|   IBIS model for TI TMS320C6474 DSP
[IBIS Ver]   5.0
[Disclaimer]   Please be aware that in the absence of a written agreement
|   Texas Instruments(TI) assumes no liability for:
|   (1) The accuracy of the IBIS models provided to your company,
|   however, the IBIS model is compliant to industry standard
|   IQ Level 2a.  Refer to IBIS Quality Section below for
|   for full details.
|   (2) The proper functioning of these Models in your design
|   or for any resulting applications
|   (3) Infringement of patents, copyrights or intellectual
|   property rights resulting from your use of these
|   models.
|   TI provides IBIS Models as a service to our customers and
|   therefore reserves the right to limit distribution of the
|   Models.  The information is subject to change without notice.
[File Name]  tms320c6474.ibs
[File Rev]   1.3
[Date]   31Mar2011
[Source]   Texas Instruments Incorporated
[Copyright]   Property of Texas Instruments Incorporated.
|   Unauthorized reproduction and/or distribution is strictly.
|   prohibited.
|   This product is protected under copyright law and trade
|   secret law as an unpublished work.
|   Created 2008,(C) Copyright 1999-2011,
|   Texas Instruments Incorporated., All Rights Reserved.
|   These commodities are under the U.S. Governmentdistribution
|   license control. As such,they are not to be re-exported without
|   the prior approval of the U.S. Department of Commerce.
[Notes]
|   Some IV curves contain Non monotonic data points.
|   The bshtltcscdvgpbfz IO buffer will exhibit a step behavior in the
|   *_SR0* mode. This behavior in the TX slow slew-rate mode is real
|   and is realized using the stage turn-on mechanism of the output
|   stage. The Tx output stage  transistor  is  composed of four equal
|   fingers and each finger is turned-on one after another. When we
|   have a resistive only load on the output, which is the case for the
|   V-t table generation, it becomes a resistive potential divider between
|   output impedance and resistive load. Since the output impedance changes
|   in four equal steps, the generated curves also reflect four equal
|   voltage steps during the rising transition. This stair stepping behavior
|   will not be seen with a capacitive load.
|   IV and VT curves generated from Quantum-SI Spice to IBIS
|   Version: 2008.06-SP1
|   Package parasitics from Optimal Corporation's PakSi-E November 09, 2006
|   Models created from the following HSPICE models:
|   - bc1825eshypdfz.hspice
|   - bc1825eshypufz.hspice
|   - bc1840dshypdfz.hspice
|   - bc1840eshyfz.hspice
|   - bc1840eshypdfz.hspice
|   - bc1850bshypdfz.hspice
|   - bc1850cshypdfz.hspice
|   - bc1850cshypufz.hspice
|   - bi2c18sfz.hspice
|   - bshtltcscdvgpbfz.hspice
|   - ic18ghy.hspice
|   - ic18shy.hspice
|   - ic18shypdfz.hspice
|   - ic18shypufz.hspice
|   - iclkrx18g.hspice
|   - ihhv18s.hspice
|   - ilvds18g.hspice
|   Revision History
|   Revision 1.3 -- 31Mar2011
|   Updated IBIS model: bshtltcscdvgpbfz
|   -added additional model selectors
|   -updated all IQ notes
|   File passes ibischk5.0.4 with 0 errors and 10 warnings.
|   -See IBIS quality notes for details.
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[Component] TMS320C6474
[Manufacturer] Texas Instruments
[Package Model] 6474
[Package]
||   Typ   Min   Max
R_pkg   0.779   0.173   1.342
L_pkg   2.688nH  1.568nH  4.416nH
C_pkg   1.455pF  1.031pF  2.178pF
[Pin] signal_name   model_name
T3   GP00   bc1825eshypdfz
U4   GP01   bc1825eshypdfz
V1   GP02   bc1825eshypdfz
U3   GP03   bc1825eshypdfz
V2   GP05   bc1825eshypdfz
V3   GP06   bc1825eshypdfz
Y3   GP07   bc1825eshypdfz
Y4   GP08   bc1825eshypdfz
AA2   GP09   bc1825eshypdfz
AA3   GP10   bc1825eshypdfz
AB4   GP11   bc1825eshypdfz
AB3   GP12   bc1825eshypdfz
AB2   GP13   bc1825eshypdfz
AA4   GP14   bc1825eshypdfz
AC3   GP15   bc1825eshypdfz
F2   TIMO0   bc1825eshypdfz
F4   TIMO1   bc1825eshypdfz
R4   EMU00   bc1825eshypufz
R2   EMU01   bc1825eshypufz
N3   EMU02   bc1825eshypufz
N1   EMU03   bc1825eshypufz
M2   EMU04   bc1825eshypufz
M1   EMU05   bc1825eshypufz
N4   EMU06   bc1825eshypufz
R3   EMU07   bc1825eshypufz
M4   EMU08   bc1825eshypufz
N2   EMU09   bc1825eshypufz
R1   EMU10   bc1825eshypufz
T2   EMU11   bc1825eshypufz
L3   EMU12   bc1825eshypufz
P4   EMU13   bc1825eshypufz
K2   EMU14   bc1825eshypufz
T1   EMU15   bc1825eshypufz
P3   EMU16   bc1825eshypufz
L4   EMU17   bc1825eshypufz
M3   EMU18   bc1825eshypufz
T4   GP04   bc1825eshypufz
B20   CLKR0   bc1840dshypdfz
A24   CLKR1   bc1840dshypdfz
C20   CLKX0   bc1840dshypdfz
C22   CLKX1   bc1840dshypdfz
D19   DX0   bc1840dshypdfz
B22   DX1   bc1840dshypdfz
B21   FSR0   bc1840dshypdfz
C21   FSR1   bc1840dshypdfz
A21   FSX0   bc1840dshypdfz
A22   FSX1   bc1840dshypdfz
AE23  DDRSLRATE   bc1840eshyfz
W3   TDO   bc1840eshyfz
AD6   SYSCLKOUT   bc1840eshypdfz
AD4   SMFRAMECLK   bc1850bshypdfz
AF6   ALTFSYNCCLK   bc1850cshypdfz
AE6   ALTFSYNCPULSE   bc1850cshypdfz
C19   MDCLK   bc1850cshypdfz
J4   NMI0   bc1850cshypdfz
J2   NMI1   bc1850cshypdfz
J1   NMI2   bc1850cshypdfz
AF4   RESETSTATz   bc1850cshypdfz
AD3   TRT   bc1850cshypdfz
AC4   TRTCLK   bc1850cshypdfz
B19   MDIO   bc1850cshypufz
E4   SCL   bi2c18sfz
D4   SDA   bi2c18sfz
G3   VCNTL0   bi2c18sfz
G2   VCNTL1   bi2c18sfz
H4   VCNTL2   bi2c18sfz
H3   VCNTL3   bi2c18sfz
K25   DDRA00   bshtltcscdvgpbfz
N25   DDRA01   bshtltcscdvgpbfz
M25   DDRA02   bshtltcscdvgpbfz
R26   DDRA03   bshtltcscdvgpbfz
L25   DDRA04   bshtltcscdvgpbfz
N27   DDRA05   bshtltcscdvgpbfz
L26   DDRA06   bshtltcscdvgpbfz
U26   DDRA07   bshtltcscdvgpbfz
K26   DDRA08   bshtltcscdvgpbfz
R27   DDRA09   bshtltcscdvgpbfz
P25   DDRA10   bshtltcscdvgpbfz
L27   DDRA11   bshtltcscdvgpbfz
U27   DDRA12   bshtltcscdvgpbfz
K27   DDRA13   bshtltcscdvgpbfz
T25   DDRBA0   bshtltcscdvgpbfz
R25   DDRBA1   bshtltcscdvgpbfz
U25   DDRBA2   bshtltcscdvgpbfz
N26   DDRCASz   bshtltcscdvgpbfz
L24   DDRCEz   bshtltcscdvgpbfz
T24   DDRCKE   bshtltcscdvgpbfz
V25   DDRCLKOUTP0   bshtltcscdvgpbfz
V24   DDRCLKOUTN0   bshtltcscdvgpbfz
J25   DDRCLKOUTP1   bshtltcscdvgpbfz
J24   DDRCLKOUTN1   bshtltcscdvgpbfz
W27   DDRD00   bshtltcscdvgpbfz
W25   DDRD01   bshtltcscdvgpbfz
Y27   DDRD02   bshtltcscdvgpbfz
W26   DDRD03   bshtltcscdvgpbfz
AA27  DDRD04   bshtltcscdvgpbfz
AA26  DDRD05   bshtltcscdvgpbfz
AA25  DDRD06   bshtltcscdvgpbfz
AA24  DDRD07   bshtltcscdvgpbfz
AC27  DDRD08   bshtltcscdvgpbfz
AC26  DDRD09   bshtltcscdvgpbfz
AC25  DDRD10   bshtltcscdvgpbfz
AD27  DDRD11   bshtltcscdvgpbfz
AC24  DDRD12   bshtltcscdvgpbfz
AE26  DDRD13   bshtltcscdvgpbfz
AE27  DDRD14   bshtltcscdvgpbfz
AE25  DDRD15   bshtltcscdvgpbfz
B25   DDRD16   bshtltcscdvgpbfz
D25   DDRD17   bshtltcscdvgpbfz
B26   DDRD18   bshtltcscdvgpbfz
D24   DDRD19   bshtltcscdvgpbfz
B27   DDRD20   bshtltcscdvgpbfz
D26   DDRD21   bshtltcscdvgpbfz
D27   DDRD22   bshtltcscdvgpbfz
C27   DDRD23   bshtltcscdvgpbfz
F24   DDRD24   bshtltcscdvgpbfz
F25   DDRD25   bshtltcscdvgpbfz
F26   DDRD26   bshtltcscdvgpbfz
F27   DDRD27   bshtltcscdvgpbfz
G27   DDRD28   bshtltcscdvgpbfz
H25   DDRD29   bshtltcscdvgpbfz
H26   DDRD30   bshtltcscdvgpbfz
H27   DDRD31   bshtltcscdvgpbfz
W24   DDRDQM0   bshtltcscdvgpbfz
AE24  DDRDQM1   bshtltcscdvgpbfz
B24   DDRDQM2   bshtltcscdvgpbfz
H24   DDRDQM3   bshtltcscdvgpbfz
Y25   DDRDQS0N   bshtltcscdvgpbfz
Y26   DDRDQS0P   bshtltcscdvgpbfz
AD25  DDRDQS1N   bshtltcscdvgpbfz
AD26  DDRDQS1P   bshtltcscdvgpbfz
C25   DDRDQS2N   bshtltcscdvgpbfz
C26   DDRDQS2P   bshtltcscdvgpbfz
G26   DDRDQS3N   bshtltcscdvgpbfz
G25   DDRDQS3P   bshtltcscdvgpbfz
K24   DDRODT   bshtltcscdvgpbfz
M24   DDRRASz   bshtltcscdvgpbfz
AB25  DDRRCVENIN0   bshtltcscdvgpbfz
E24   DDRRCVENIN1   bshtltcscdvgpbfz
AB24  DDRRCVENOUT0   bshtltcscdvgpbfz
E25   DDRRCVENOUT1   bshtltcscdvgpbfz
P24   DDRWEz   bshtltcscdvgpbfz
AF7   CORECLKSEL   ic18ghy
AD5   XWRSTz   ic18shy
D20   CLKS0   ic18shypdfz
A25   CLKS1   ic18shypdfz
A20   DR0   ic18shypdfz
D21   DR1   ic18shypdfz
E3   TIMI0   ic18shypdfz
C4   TIMI1   ic18shypdfz
W2   TRSTz   ic18shypdfz
W4   TCK   ic18shypufz
V4   TDI   ic18shypufz
W1   TMS   ic18shypufz
AF9   ALTCORECLKP   iclkrx18g
AF10  ALTCORECLKN   iclkrx18g
AD24  DDRREFCLKP   iclkrx18g
AD23  DDRREFCLKN   iclkrx18g
C9   RIOSGMIICLKP   iclkrx18g
D9   RIOSGMIICLKN   iclkrx18g
AE9   SYSCLKP   iclkrx18g
AE10  SYSCLKN   iclkrx18g
AE5   PORz   ihhv18s
AD9   FRAMEBURSTP   ilvds18g
AD10  FRAMEBURSTN   ilvds18g
AD7   FSYNCCLKP   ilvds18g
AD8   FSYNCCLKN   ilvds18g
C16   SGMII_RXN0   NC
C17   SGMII_RXP0   NC
A16   SGMII_TXN0   NC
A15   SGMII_TXP0   NC
C11   RIOTXN0   NC
C10   RIOTXP0   NC
C13   RIOTXN1   NC
C14   RIOTXP1   NC
A9   RIORXN0   NC
A10   RIORXP0   NC
A13   RIORXN1   NC
A12   RIORXP1   NC
AE19  RSV01   NC
AD14  RSV02   NC
N24   RSV03   NC
AG10  RSV04   NC
AG24  RSV05   NC
AE7   RSV06   NC
AE8   RSV07   NC
AF24  RSV08   NC
AF25  RSV09   NC
K4   RSV10   bc1825eshypufz
K3   RSV11   bc1825eshypufz
K1   RSV12   bc1825eshypufz
G4   RSV13   bc1850bshypdfz
F3   RSV14   bc1850bshypdfz
D7   RSV15   NC
C7   RSV16   NC
B12   RSV17   NC
B18   RSV18   NC
D6   RSV19   bc1825eshypufz
C6   RSV20   bc1825eshypufz
E6   RSV21   NC
E7   RSV22   NC
AE4   RSV23   bc1850cshypdfz
AG25  RSV24   bc1850cshypdfz
D22   RSV25   NC
C23   RSV26   NC
D5   RSV27   NC
C5   RSV28   NC
J3   RSV29   ic18shypufz
AF22  AIFRXN0   NC
AF21  AIFRXP0   NC
AG20  AIFRXN1   NC
AG21  AIFRXP1   NC
AG18  AIFRXN2   NC
AG17  AIFRXP2   NC
AE17  AIFRXN3   NC
AE18  AIFRXP3   NC
AE14  AIFRXN4   NC
AE13  AIFRXP4   NC
AF12  AIFRXN5   NC
AF13  AIFRXP5   NC
AE21  AIFTXN0   NC
AE22  AIFTXP0   NC
AD21  AIFTXN1   NC
AD20  AIFTXP1   NC
AF16  AIFTXN2   NC
AF17  AIFTXP2   NC
AD17  AIFTXN3   NC
AD16  AIFTXP3   NC
AG13  AIFTXN4   NC
AG14  AIFTXP4   NC
AD13  AIFTXN5   NC
AD12  AIFTXP5   NC
T26   VREFSSTL   POWER
J11   CVdd   POWER
J17   CVdd   POWER
J19   CVdd   POWER
J9   CVdd   POWER
K10   CVdd   POWER
K18   CVdd   POWER
L11   CVdd   POWER
L13   CVdd   POWER
L15   CVdd   POWER
L17   CVdd   POWER
L19   CVdd   POWER
L9   CVdd   POWER
M10   CVdd   POWER
M12   CVdd   POWER
M14   CVdd   POWER
M16   CVdd   POWER
M18   CVdd   POWER
N11   CVdd   POWER
N13   CVdd   POWER
N15   CVdd   POWER
N17   CVdd   POWER
N19   CVdd   POWER
N9   CVdd   POWER
P10   CVdd   POWER
P12   CVdd   POWER
P14   CVdd   POWER
P16   CVdd   POWER
P18   CVdd   POWER
R11   CVdd   POWER
R13   CVdd   POWER
R15   CVdd   POWER
R17   CVdd   POWER
R19   CVdd   POWER
R9   CVdd   POWER
T10   CVdd   POWER
T12   CVdd   POWER
T14   CVdd   POWER
T16   CVdd   POWER
T18   CVdd   POWER
U11   CVdd   POWER
U13   CVdd   POWER
U15   CVdd   POWER
U19   CVdd   POWER
U9   CVdd   POWER
V10   CVdd   POWER
V12   CVdd   POWER
V14   CVdd   POWER
W11   CVdd   POWER
W13   CVdd   POWER
W9   CVdd   POWER
AG26  AIF_VDDD11   POWER
U17   AIF_VDDD11   POWER
V16   AIF_VDDD11   POWER
V18   AIF_VDDD11   POWER
W15   AIF_VDDD11   POWER
W17   AIF_VDDD11   POWER
W19   AIF_VDDD11   POWER
D12   SGR_VDDA11   POWER
D18   SGR_VDDA11   POWER
E11   SGR_VDDA11   POWER
E15   SGR_VDDA11   POWER
AG23  AVDD218   POWER
AG9   AVDD118   POWER
AC12  AIF_VDDA11   POWER
AC15  AIF_VDDA11   POWER
AC18  AIF_VDDA11   POWER
AC21  AIF_VDDA11   POWER
J13   SGR_VDDD11   POWER
J15   SGR_VDDD11   POWER
K12   SGR_VDDD11   POWER
K14   SGR_VDDD11   POWER
K16   SGR_VDDD11   POWER
AG6   CVDDMON   POWER
C12   SGR_VDDR18   POWER
A18   SGR_VDDR18   POWER
AD19  AIF_VDDR18   POWER
AD15  AIF_VDDR18   POWER
A1   DVDD18   POWER
A19   DVDD18   POWER
A23   DVDD18   POWER
A27   DVDD18   POWER
A5   DVDD18   POWER
AA23  DVDD18   POWER
AA5   DVDD18   POWER
AB26  DVDD18   POWER
AC1   DVDD18   POWER
AC23  DVDD18   POWER
AC5   DVDD18   POWER
AC7   DVDD18   POWER
AC9   DVDD18   POWER
AF5   DVDD18   POWER
AG1   DVDD18   POWER
AG27  DVDD18   POWER
AG8   DVDD18   POWER
E1   DVDD18   POWER
E19   DVDD18   POWER
E21   DVDD18   POWER
E23   DVDD18   POWER
E27   DVDD18   POWER
E5   DVDD18   POWER
G23   DVDD18   POWER
G5   DVDD18   POWER
H2   DVDD18   POWER
J23   DVDD18   POWER
J27   DVDD18   POWER
J5   DVDD18   POWER
L1   DVDD18   POWER
L23   DVDD18   POWER
L5   DVDD18   POWER
M26   DVDD18   POWER
N23   DVDD18   POWER
N5   DVDD18   POWER
P2   DVDD18   POWER
P26   DVDD18   POWER
R23   DVDD18   POWER
R5   DVDD18   POWER
U1   DVDD18   POWER
U23   DVDD18   POWER
U5   DVDD18   POWER
V26   DVDD18   POWER
W23   DVDD18   POWER
W5   DVDD18   POWER
Y2   DVDD18   POWER
Y24   DVDD18   POWER
AG7   DVDD18MON   POWER
B13   SGR_VDDT11   POWER
B17   SGR_VDDT11   POWER
B8   SGR_VDDT11   POWER
E13   SGR_VDDT11   POWER
E17   SGR_VDDT11   POWER
E9   SGR_VDDT11   POWER
AC11  AIF_VDDT11   POWER
AC14  AIF_VDDT11   POWER
AC17  AIF_VDDT11   POWER
AC20  AIF_VDDT11   POWER
AF15  AIF_VDDT11   POWER
AF19  AIF_VDDT11   POWER
AG11  AIF_VDDT11   POWER
A11   VSS   GND
A14   VSS   GND
A17   VSS   GND
A2   VSS   GND
A26   VSS   GND
A3   VSS   GND
A4   VSS   GND
A6   VSS   GND
A7   VSS   GND
A8   VSS   GND
AA1   VSS   GND
AB1   VSS   GND
AB23  VSS   GND
AB27  VSS   GND
AB5   VSS   GND
AC10  VSS   GND
AC13  VSS   GND
AC16  VSS   GND
AC19  VSS   GND
AC2   VSS   GND
AC22  VSS   GND
AC6   VSS   GND
AC8   VSS   GND
AD1   VSS   GND
AD11  VSS   GND
AD18  VSS   GND
AD2   VSS   GND
AD22  VSS   GND
AE1   VSS   GND
AE11  VSS   GND
AE12  VSS   GND
AE15  VSS   GND
AE16  VSS   GND
AE2   VSS   GND
AE20  VSS   GND
AE3   VSS   GND
AF1   VSS   GND
AF11  VSS   GND
AF14  VSS   GND
AF18  VSS   GND
AF2   VSS   GND
AF20  VSS   GND
AF23  VSS   GND
AF26  VSS   GND
AF27  VSS   GND
AF3   VSS   GND
AF8   VSS   GND
AG12  VSS   GND
AG15  VSS   GND
AG16  VSS   GND
AG19  VSS   GND
AG2   VSS   GND
AG22  VSS   GND
AG3   VSS   GND
AG4   VSS   GND
AG5   VSS   GND
B1   VSS   GND
B10   VSS   GND
B11   VSS   GND
B14   VSS   GND
B15   VSS   GND
B16   VSS   GND
B2   VSS   GND
B23   VSS   GND
B3   VSS   GND
B4   VSS   GND
B5   VSS   GND
B6   VSS   GND
B7   VSS   GND
B9   VSS   GND
C1   VSS   GND
C15   VSS   GND
C18   VSS   GND
C2   VSS   GND
C24   VSS   GND
C3   VSS   GND
C8   VSS   GND
D1   VSS   GND
D10   VSS   GND
D11   VSS   GND
D13   VSS   GND
D14   VSS   GND
D15   VSS   GND
D16   VSS   GND
D17   VSS   GND
D2   VSS   GND
D23   VSS   GND
D3   VSS   GND
D8   VSS   GND
E10   VSS   GND
E12   VSS   GND
E14   VSS   GND
E16   VSS   GND
E18   VSS   GND
E2   VSS   GND
E20   VSS   GND
E22   VSS   GND
E26   VSS   GND
E8   VSS   GND
F1   VSS   GND
F23   VSS   GND
F5   VSS   GND
G1   VSS   GND
G24   VSS   GND
H1   VSS   GND
H23   VSS   GND
H5   VSS   GND
J10   VSS   GND
J12   VSS   GND
J14   VSS   GND
J16   VSS   GND
J18   VSS   GND
J26   VSS   GND
K11   VSS   GND
K13   VSS   GND
K15   VSS   GND
K17   VSS   GND
K19   VSS   GND
K23   VSS   GND
K5   VSS   GND
K9   VSS   GND
L10   VSS   GND
L12   VSS   GND
L14   VSS   GND
L16   VSS   GND
L18   VSS   GND
L2   VSS   GND
M11   VSS   GND
M13   VSS   GND
M15   VSS   GND
M17   VSS   GND
M19   VSS   GND
M23   VSS   GND
M27   VSS   GND
M5   VSS   GND
M9   VSS   GND
N10   VSS   GND
N12   VSS   GND
N14   VSS   GND
N16   VSS   GND
N18   VSS   GND
P1   VSS   GND
P11   VSS   GND
P13   VSS   GND
P15   VSS   GND
P17   VSS   GND
P19   VSS   GND
P23   VSS   GND
P27   VSS   GND
P5   VSS   GND
P9   VSS   GND
R10   VSS   GND
R12   VSS   GND
R14   VSS   GND
R16   VSS   GND
R18   VSS   GND
R24   VSS   GND
T11   VSS   GND
T13   VSS   GND
T15   VSS   GND
T17   VSS   GND
T19   VSS   GND
T23   VSS   GND
T27   VSS   GND
T5   VSS   GND
T9   VSS   GND
U10   VSS   GND
U12   VSS   GND
U14   VSS   GND
U16   VSS   GND
U18   VSS   GND
U2   VSS   GND
U24   VSS   GND
V11   VSS   GND
V13   VSS   GND
V15   VSS   GND
V17   VSS   GND
V19   VSS   GND
V23   VSS   GND
V27   VSS   GND
V5   VSS   GND
V9   VSS   GND
W10   VSS   GND
W12   VSS   GND
W14   VSS   GND
W16   VSS   GND
W18   VSS   GND
Y1   VSS   GND
Y23   VSS   GND
Y5   VSS   GND
|********************  DIFF PIN  *******************************
[Diff_pin]   inv_pin   vdiff  tdelay_typ  tdelay_min  tdelay_max
|V25   V24   NA   NA   NA   NA   || DDRCLKOUTP0 DDRCLKOUTN0
|J25   J24   NA   NA   NA   NA   || DDRCLKOUTP1 DDRCLKOUTN1
|Y26   Y25   NA   NA   NA   NA   || DDRDQS0P DDRDQS0N
|AD26   AD25   NA   NA   NA   NA   || DDRDQS1P DDRDQS1N
|C26   C25   NA   NA   NA   NA   || DDRDQS2P DDRDQS2N
|G25   G26   NA   NA   NA   NA   || DDRDQS3P DDRDQS3N
AF9   AF10   0.100  NA   NA   NA   || ALTCORECLKP ALTCORECLKN
AD24   AD23   0.100  NA   NA   NA   || DDRREFCLKP DDRREFCLKN
C9   D9   0.100  NA   NA   NA   || RIOSGMIICLKP RIOSGMIICLKN
AE9   AE10   0.100  NA   NA   NA   || SYSCLKP SYSCLKN
AD9   AD10   0.100  NA   NA   NA   || FRAMEBURSTP FRAMEBURSTN
AD7   AD8   0.100  NA   NA   NA   || FSYNCCLKP FSYNCCLKN
|   Component BSHTLTCSCDVGPBFZ
[Model Selector] bshtltcscdvgpbfz
|   -The designation "SR" refers to Slew Rate
|   -The designation 1p8" refers to 1.8 where "p" refers to "point"
|   -The designation "NOSR" refers to No Slew Rate
|   -The designation "10PER" refers to 10 percent
|   -The designation "NOTERM" refers to no thevenin termination
|   -The designation "HALFTERM" refers to half thevenin termination
|   -The designation "FULLTERM" refers to full thevenin termination
NOSR0_10PER_45OHM_1P8  TX MODE,1.8V +/- 10PERCENT,45OHM,FAST SLEWRATE (SR0=0)
|NOSR0_10PER_45OHM_1P8;
SR0_10PER_45OHM_1P8  TX MODE,1.8V +/- 10PERCENT,45OHM,SLOW SLEWRATE (SR0=1)
|SR0_10PER_45OHM_1P8;
NOSR0_5PER_45OHM_1P8  TX MODE,1.8V +/- 5PERCENT,45OHM,FAST SLEWRATE (SR0=0)
|NOSR0_5PER_45OHM_1P8;
SR0_5PER_45OHM_1P8  TX MODE,1.8V +/- 5PERCENT,45OHM,SLOW SLEWRATE (SR0=1)
|SR0_5PER_45OHM_1P8;
NOSR0_10PER_50OHM_1P8  TX MODE,1.8V +/- 10PERCENT,50OHM,FAST SLEWRATE (SR0=0)
|NOSR0_10PER_50OHM_1P8;
SR0_10PER_50OHM_1P8  TX MODE,1.8V +/- 10PERCENT,50OHM,SLOW SLEWRATE (SR0=1)
|SR0_10PER_50OHM_1P8;
NOSR0_5PER_50OHM_1P8  TX MODE,1.8V +/- 5PERCENT,50OHM,FAST SLEWRATE (SR0=0)
|NOSR0_5PER_50OHM_1P8;
SR0_5PER_50OHM_1P8  TX MODE,1.8V +/- 5PERCENT,50OHM,SLOW SLEWRATE (SR0=1)
|SR0_5PER_50OHM_1P8;
NOSR0_10PER_55OHM_1P8  TX MODE,1.8V +/- 10PERCENT,55OHM,FAST SLEWRATE (SR0=0)
|NOSR0_10PER_55OHM_1P8;
SR0_10PER_55OHM_1P8  TX MODE,1.8V +/- 10PERCENT,55OHM,SLOW SLEWRATE (SR0=1)
|SR0_10PER_55OHM_1P8;
NOSR0_5PER_55OHM_1P8  TX MODE,1.8V +/- 5PERCENT,55OHM,FAST SLEWRATE (SR0=0)
|NOSR0_5PER_55OHM_1P8;
SR0_5PER_55OHM_1P8  TX MODE,1.8V +/- 5PERCENT,55OHM,SLOW SLEWRATE (SR0=1)
|SR0_5PER_55OHM_1P8;
NOSR0_10PER_30OHM_1P8  TX MODE,1.8V +/- 10PERCENT,30OHM,FAST SLEWRATE (SR0=0)
|NOSR0_10PER_30OHM_1P8;
SR0_10PER_30OHM_1P8  TX MODE,1.8V +/- 10PERCENT,30OHM,SLOW SLEWRATE (SR0=1)
|SR0_10PER_30OHM_1P8;
NOSR0_5PER_30OHM_1P8  TX MODE,1.8V +/- 5PERCENT,30OHM,FAST SLEWRATE (SR0=0)
|NOSR0_5PER_30OHM_1P8;
SR0_5PER_30OHM_1P8  TX MODE,1.8V +/- 5PERCENT,30OHM,SLOW SLEWRATE (SR0=1)
|SR0_5PER_30OHM_1P8;
45OHM_10PER_HALFTERM_1P8  RX MODE,1.8V +/- 10PERCENT,90OHM ON DIE TERMINATION
|45OHM_10PER_HALFTERM_1P8;
45OHM_10PER_NOTERM_1P8  RX MODE,1.8V +/- 10PERCENT,WITHOUT TERMINATION
|45OHM_10PER_NOTERM_1P8;
45OHM_10PER_FULLTERM_1P8  RX MODE,1.8V +/- 10PERCENT,45OHM ON DIE TERMINATION
|45OHM_10PER_FULLTERM_1P8;
45OHM_5PER_HALFTERM_1P8  RX MODE,1.8V +/- 5PERCENT,90OHM ON DIE TERMINATION
|45OHM_5PER_HALFTERM_1P8;
45OHM_5PER_NOTERM_1P8  RX MODE,1.8V +/- 5PERCENT,WITHOUT TERMINATION
|45OHM_5PER_NOTERM_1P8;
45OHM_5PER_FULLTERM_1P8  RX MODE,1.8V +/- 5PERCENT,45OHM ON DIE TERMINATION
|45OHM_5PER_FULLTERM_1P8;
50OHM_10PER_HALFTERM_1P8  RX MODE,1.8V +/- 10PERCENT,100OHM ON DIE TERMINATION
|50OHM_10PER_HALFTERM_1P8;
50OHM_10PER_NOTERM_1P8  RX MODE,1.8V +/- 10PERCENT,WITHOUT TERMINATION
|50OHM_10PER_NOTERM_1P8;
50OHM_10PER_FULLTERM_1P8  RX MODE,1.8V +/- 10PERCENT,50OHM ON DIE TERMINATION
|50OHM_10PER_FULLTERM_1P8;
50OHM_5PER_HALFTERM_1P8  RX MODE,1.8V +/- 5PERCENT,100OHM ON DIE TERMINATION
|50OHM_5PER_HALFTERM_1P8;
50OHM_5PER_NOTERM_1P8  RX MODE,1.8V +/- 5PERCENT,WITHOUT TERMINATION
|50OHM_5PER_NOTERM_1P8;
50OHM_5PER_FULLTERM_1P8  RX MODE,1.8V +/- 5PERCENT,50OHM ON DIE TERMINATION
|50OHM_5PER_FULLTERM_1P8;
55OHM_10PER_HALFTERM_1P8  RX MODE,1.8V +/- 10PERCENT,110OHM ON DIE TERMINATION
|55OHM_10PER_HALFTERM_1P8;
55OHM_10PER_NOTERM_1P8  RX MODE,1.8V +/- 10PERCENT,WITHOUT TERMINATION
|55OHM_10PER_NOTERM_1P8;
55OHM_10PER_FULLTERM_1P8  RX MODE,1.8V +/- 10PERCENT,55OHM ON DIE TERMINATION
|55OHM_10PER_FULLTERM_1P8;
55OHM_5PER_HALFTERM_1P8  RX MODE,1.8V +/- 5PERCENT,110OHM ON DIE TERMINATION
|55OHM_5PER_HALFTERM_1P8;
55OHM_5PER_NOTERM_1P8  RX MODE,1.8V +/- 5PERCENT,WITHOUT TERMINATION
|55OHM_5PER_NOTERM_1P8;
55OHM_5PER_FULLTERM_1P8  RX MODE,1.8V +/- 5PERCENT,55OHM ON DIE TERMINATION
|55OHM_5PER_FULLTERM_1P8;
30OHM_10PER_HALFTERM_1P8  RX MODE,1.8V +/- 10PERCENT,60OHM ON DIE TERMINATION
|30OHM_10PER_HALFTERM_1P8;
30OHM_10PER_NOTERM_1P8  RX MODE,1.8V +/- 10PERCENT,WITHOUT TERMINATION
|30OHM_10PER_NOTERM_1P8;
30OHM_10PER_FULLTERM_1P8  RX MODE,1.8V +/- 10PERCENT,30OHM ON DIE TERMINATION
|30OHM_10PER_FULLTERM_1P8;
30OHM_5PER_HALFTERM_1P8  RX MODE,1.8V +/- 5PERCENT,60OHM ON DIE TERMINATION
|30OHM_5PER_HALFTERM_1P8;
30OHM_5PER_NOTERM_1P8  RX MODE,1.8V +/- 5PERCENT,WITHOUT TERMINATION
|30OHM_5PER_NOTERM_1P8;
30OHM_5PER_FULLTERM_1P8  RX MODE,1.8V +/- 5PERCENT,30OHM ON DIE TERMINATION
|   Package Model Definition
[Define Package Model]  6474
[Manufacturer]   Texas Instruments Incorporated
[OEM]   Texas Instruments Incorporated
[Description]   6474 pkg with all signals except SERDES
[Number Of Pins]   203
[Pin Numbers]
G27   | 1   G27   DDR_DATA[28]
H26   | 2   H26   DDR_DATA[30]
F27   | 3   F27   DDR_DATA[27]
F25   | 4   F25   DDR_DATA[25]
F26   | 5   F26   DDR_DATA[26]
F24   | 6   F24   DDR_DATA[24]
H25   | 7   H25   DDR_DATA[29]
H27   | 8   H27   DDR_DATA[31]
B27   | 9   B27   DDR_DATA[20]
D27   | 10   D27   DDR_DATA[22]
D24   | 11   D24   DDR_DATA[19]
D25   | 12   D25   DDR_DATA[17]
B26   | 13   B26   DDR_DATA[18]
B25   | 14   B25   DDR_DATA[16]
D26   | 15   D26   DDR_DATA[21]
C27   | 16   C27   DDR_DATA[23]
AE26   | 17   AE26   DDR_DATA[13]
AE25   | 18   AE25   DDR_DATA[15]
AC24   | 19   AC24   DDR_DATA[12]
AE27   | 20   AE27   DDR_DATA[14]
AD27   | 21   AD27   DDR_DATA[11]
AC26   | 22   AC26   DDR_DATA[9]
AC25   | 23   AC25   DDR_DATA[10]
AC27   | 24   AC27   DDR_DATA[8]
Y27   | 25   Y27   DDR_DATA[2]
W27   | 26   W27   DDR_DATA[0]
AA26   | 27   AA26   DDR_DATA[5]
AA24   | 28   AA24   DDR_DATA[7]
AA27   | 29   AA27   DDR_DATA[4]
AA25   | 30   AA25   DDR_DATA[6]
W25   | 31   W25   DDR_DATA[1]
W26   | 32   W26   DDR_DATA[3]
T26   | 33   T26   VREFHSTL
C6   | 34   C6   RSV20
D6   | 35   D6   RSV19
AF9   | 36   AF9   ALT_CORE_CLK_P
AF10   | 37   AF10   ALT_CORE_CLK_N
AD5   | 38   AD5   XWRST_L
J3   | 39   J3   RSV29
H3   | 40   H3   VCNTL[3]
H4   | 41   H4   VCNTL[2]
G2   | 42   G2   VCNTL[1]
G3   | 43   G3   VCNTL[0]
AE6   | 44   AE6   UMTS_SYNC
AF6   | 45   AF6   UMTS_CLK
AC4   | 46   AC4   TRT_CLK
AD3   | 47   AD3   TRT
W2   | 48   W2   TRST
W1   | 49   W1   TMS
F4   | 50   F4   TIMERO[1]
F2   | 51   F2   TIMERO[0]
C4   | 52   C4   TIMERI[1]
E3   | 53   E3   TIMERI[0]
C23   | 54   C23   RSV26
C5   | 55   C5   RSV28
D22   | 56   D22   RSV25
D5   | 57   D5   RSV27
W3   | 58   W3   TDO
V4   | 59   V4   TDI
W4   | 60   W4   TCK
AD6   | 61   AD6   SYSCLKOUT_CLK
AE9   | 62   AE9   SYS_AI_CORE_CLK_P
AE10   | 63   AE10   SYS_AI_CORE_CLK_N
C9   | 64   C9   SRIO_SGMII_CLK_P
D9   | 65   D9   SRIO_SGMII_CLK_N
AD4   | 66   AD4   SM_FRAME_CLK
AF4   | 67   AF4   RESET_STATUS_N
AE5   | 68   AE5   POR_L
C7   | 69   C7   RSV16
D7   | 70   D7   RSV15
J1   | 71   J1   NMI[2]
J2   | 72   J2   NMI[1]
J4   | 73   J4   NMI[0]
A22   | 74   A22   MCBSP_FSX[1]
A21   | 75   A21   MCBSP_FSX[0]
C21   | 76   C21   MCBSP_FSR[1]
B21   | 77   B21   MCBSP_FSR[0]
B22   | 78   B22   MCBSP_DATAX[1]
D19   | 79   D19   MCBSP_DATAX[0]
D21   | 80   D21   MCBSP_DATAR[1]
A20   | 81   A20   MCBSP_DATAR[0]
C22   | 82   C22   MCBSP_CLKX[1]
C20   | 83   C20   MCBSP_CLKX[0]
A25   | 84   A25   MCBSP_CLKS[1]
D20   | 85   D20   MCBSP_CLKS[0]
A24   | 86   A24   MCBSP_CLKR[1]
B20   | 87   B20   MCBSP_CLKR[0]
D4   | 88   D4   I2C_SDA
E4   | 89   E4   I2C_SCL
AA2   | 90   AA2   GPIO[9]
Y4   | 91   Y4   GPIO[8]
Y3   | 92   Y3   GPIO[7]
V3   | 93   V3   GPIO[6]
V2   | 94   V2   GPIO[5]
T4   | 95   T4   GPIO[4]
U3   | 96   U3   GPIO[3]
V1   | 97   V1   GPIO[2]
AC3   | 98   AC3   GPIO[15]
AA4   | 99   AA4   GPIO[14]
AB2   | 100   AB2   GPIO[13]
AB3   | 101   AB3   GPIO[12]
AB4   | 102   AB4   GPIO[11]
AA3   | 103   AA3   GPIO[10]
U4   | 104   U4   GPIO[1]
T3   | 105   T3   GPIO[0]
AD7   | 106   AD7   FSYNC_CLK_P
AD8   | 107   AD8   FSYNC_CLK_N
AD9   | 108   AD9   FRAME_BURST_P
AD10   | 109   AD10   FRAME_BURST_N
F3   | 110   F3   RSV14
G4   | 111   G4   RSV13
B19   | 112   B19   ETHERNET_MDIO_DATA
C19   | 113   C19   ETHERNET_MDIO_CLK
N2   | 114   N2   EMU[9]
M4   | 115   M4   EMU[8]
R3   | 116   R3   EMU[7]
N4   | 117   N4   EMU[6]
M1   | 118   M1   EMU[5]
M2   | 119   M2   EMU[4]
N1   | 120   N1   EMU[3]
K1   | 121   K1   RSV12
K3   | 122   K3   RSV11
N3   | 123   N3   EMU[2]
K4   | 124   K4   RSV10
M3   | 125   M3   EMU[18]
L4   | 126   L4   EMU[17]
P3   | 127   P3   EMU[16]
T1   | 128   T1   EMU[15]
K2   | 129   K2   EMU[14]
P4   | 130   P4   EMU[13]
L3   | 131   L3   EMU[12]
T2   | 132   T2   EMU[11]
R1   | 133   R1   EMU[10]
R2   | 134   R2   EMU[1]
R4   | 135   R4   EMU[0]
AE7   | 136   AE7   RSV06
AE8   | 137   AE8   RSV07
AE4   | 138   AE4   RSV23
AG10   | 139   AG10   RSV04
AF7   | 140   AF7   ALT_CORE_CLK_SEL
AE23   | 141   AE23   DDRSLRATE
AF24   | 142   AF24   RSV08
AF25   | 143   AF25   RSV09
AG25   | 144   AG25   RSV24
AG24   | 145   AG24   RSV05
AD24   | 146   AD24   DDR_REFCLK_CLK_P
AD23   | 147   AD23   DDR_REFCLK_CLK_N
A15   | 148   A15   SGMII_TXP0
A16   | 149   A16   SGMII_TXN0
C17   | 150   C17   SGMII_RXP0
C16   | 151   C16   SGMII_RXN0
C14   | 152   C14   SRIO_TXP1
C10   | 153   C10   SRIO_TXP0
C13   | 154   C13   SRIO_TXN1
C11   | 155   C11   SRIO_TXN0
A12   | 156   A12   SRIO_RXP1
A10   | 157   A10   SRIO_RXP0
A13   | 158   A13   SRIO_RXN1
A9   | 159   A9   SRIO_RXN0
N24   | 160   N24   RSV03
P24   | 161   P24   DDR_SDWE_L
M24   | 162   M24   DDR_SDRAS_L
T24   | 163   T24   DDR_SDCKE
N26   | 164   N26   DDR_SDCAS_L
K24   | 165   K24   DDR_ODT[0]
E25   | 166   E25   DDR_MSTRBEN_OUT[1]
AB24   | 167   AB24   DDR_MSTRBEN_OUT[0]
E24   | 168   E24   DDR_MSTRBEN_IN[1]
AB25   | 169   AB25   DDR_MSTRBEN_IN[0]
G25   | 170   G25   DDR_DQS_P[3]
C26   | 171   C26   DDR_DQS_P[2]
AD26   | 172   AD26   DDR_DQS_P[1]
Y26   | 173   Y26   DDR_DQS_P[0]
G26   | 174   G26   DDR_DQS_N[3]
C25   | 175   C25   DDR_DQS_N[2]
AD25   | 176   AD25   DDR_DQS_N[1]
Y25   | 177   Y25   DDR_DQS_N[0]
H24   | 178   H24   DDR_DQM[3]
B24   | 179   B24   DDR_DQM[2]
AE24   | 180   AE24   DDR_DQM[1]
W24   | 181   W24   DDR_DQM[0]
L24   | 182   L24   DDR_CS
J25   | 183   J25   DDR_CLK_P[1]
V25   | 184   V25   DDR_CLK_P[0]
J24   | 185   J24   DDR_CLK_N[1]
V24   | 186   V24   DDR_CLK_N[0]
U25   | 187   U25   DDR_BA[2]
R25   | 188   R25   DDR_BA[1]
T25   | 189   T25   DDR_BA[0]
R27   | 190   R27   DDR_A[9]
K26   | 191   K26   DDR_A[8]
U26   | 192   U26   DDR_A[7]
L26   | 193   L26   DDR_A[6]
N27   | 194   N27   DDR_A[5]
L25   | 195   L25   DDR_A[4]
R26   | 196   R26   DDR_A[3]
M25   | 197   M25   DDR_A[2]
K27   | 198   K27   DDR_A[13]
U27   | 199   U27   DDR_A[12]
L27   | 200   L27   DDR_A[11]
P25   | 201   P25   DDR_A[10]
N25   | 202   N25   DDR_A[1]
K25   | 203   K25   DDR_A[0]
[Model Data]
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[End Model Data]
[End Package Model]
| Models and submodels in the file (56): bc1825eshypdfz (I/O), bc1825eshypufz (I/O), bc1840dshypdfz (I/O), bc1840eshyfz (I/O), bc1840eshypdfz (I/O), bc1850bshypdfz (I/O), bc1850cshypdfz (I/O), bc1850cshypufz (I/O), NOSR0_10PER_45OHM_1P8 (3-state), SR0_10PER_45OHM_1P8 (3-state), NOSR0_5PER_45OHM_1P8 (3-state), SR0_5PER_45OHM_1P8 (3-state), NOSR0_10PER_50OHM_1P8 (3-state), SR0_10PER_50OHM_1P8 (3-state), NOSR0_5PER_50OHM_1P8 (3-state), SR0_5PER_50OHM_1P8 (3-state), NOSR0_10PER_55OHM_1P8 (3-state), SR0_10PER_55OHM_1P8 (3-state), NOSR0_5PER_55OHM_1P8 (3-state), SR0_5PER_55OHM_1P8 (3-state), NOSR0_10PER_30OHM_1P8 (3-state), SR0_10PER_30OHM_1P8 (3-state), NOSR0_5PER_30OHM_1P8 (3-state), SR0_5PER_30OHM_1P8 (3-state), 45OHM_10PER_HALFTERM_1P8 (Input), 45OHM_10PER_NOTERM_1P8 (Input), 45OHM_10PER_FULLTERM_1P8 (Input), 45OHM_5PER_HALFTERM_1P8 (Input), 45OHM_5PER_NOTERM_1P8 (Input), 45OHM_5PER_FULLTERM_1P8 (Input), 50OHM_10PER_HALFTERM_1P8 (Input), 50OHM_10PER_NOTERM_1P8 (Input), 50OHM_10PER_FULLTERM_1P8 (Input), 50OHM_5PER_HALFTERM_1P8 (Input), 50OHM_5PER_NOTERM_1P8 (Input), 50OHM_5PER_FULLTERM_1P8 (Input), 55OHM_10PER_HALFTERM_1P8 (Input), 55OHM_10PER_NOTERM_1P8 (Input), 55OHM_10PER_FULLTERM_1P8 (Input), 55OHM_5PER_HALFTERM_1P8 (Input), 55OHM_5PER_NOTERM_1P8 (Input), 55OHM_5PER_FULLTERM_1P8 (Input), 30OHM_10PER_HALFTERM_1P8 (Input), 30OHM_10PER_NOTERM_1P8 (Input), 30OHM_10PER_FULLTERM_1P8 (Input), 30OHM_5PER_HALFTERM_1P8 (Input), 30OHM_5PER_NOTERM_1P8 (Input), 30OHM_5PER_FULLTERM_1P8 (Input), ic18shy (Input), ic18shypufz (Input), ic18shypdfz (Input), ic18ghy (Input), ihhv18s (Input), bi2c18sfz (I/O_open_drain), ilvds18g (Input), iclkrx18g (Input)
